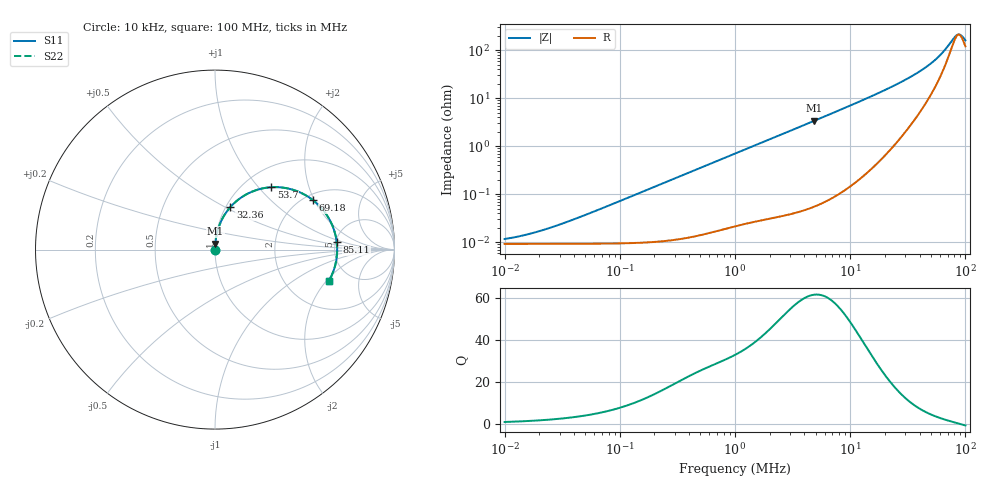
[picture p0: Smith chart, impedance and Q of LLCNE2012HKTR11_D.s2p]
! LLCNE2012HKTR11_D  S-PARAMETER MODEL  ( Standard Model )
! Model Generated by TAIYO YUDEN Corporation (http://www.ty-top.com)
! Version 1.0
! TAIYO YUDEN Control No. 210402
! Copyright(c) 2021 TAIYO YUDEN CO.,LTD. All Rights Reserved.
! Product Description (link to TY-COMPAS)
! https://ds.yuden.co.jp/TYCOMPAS/or/detail?pn=LLCNE2012HKTR11MD&u=M
! Products Name : Inductors
! Characteristics :
!  Inductance : 0.11 [uH] , SRF(min) : - [Hz] , DC Resistance(max) : 12 [mOhm]
!  Rated Current : Saturation  6.9 [A] (dL = 30 [%]), Temp Rise  5.8 [A] (dT = 40 [degC])
!  Case Size : 2.0 x 1.25 / 0.079 x 0.049 [mm/inch] , Thickness : 0.8 / 0.031 [mm/inch]
!  (Conditions: Temperature = 25 [degC] , DC Bias Current = 0 [A])
! External Node Assignments :
!  1  o---GGG---o  2
! GND o---------o GND
! Frequency Range : 10kHz  -  100MHz  [ 402 STEP ]
# MHz S RI R 50
! Freq[MHz].  S11 Real  S11 Imag  S21 Real  S21 Imag  S12 Real  S12 Imag  S22 Real  S22 Imag
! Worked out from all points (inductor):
!   401 points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, 10 kHz to 100 MHz, reference 50 ohm
!   read as one part in series: L = 113 nH near 38.91 kHz
!   highest Q = 61.6 at 4.898 MHz (marker M1), where L = 111 nH
!   self-resonance near 87.6 MHz
!   S11 on the Smith chart (normalised r, x): 10 kHz: 1.00, +0.00; 32.36 MHz: 1.05, +0.53; 53.7 MHz: 1.32, +1.17; 69.18 MHz: 2.22, +1.95; 85.11 MHz: 5.12, +0.78; 100 MHz: 3.41, -2.13
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0.01  9.2e-05 7.13e-05  0.9999 -7.13e-05  0.9999 -7.13e-05  9.2e-05 7.13e-05
0.013804  9.2e-05 9.84e-05  0.9999 -9.84e-05  0.9999 -9.84e-05  9.2e-05 9.84e-05
0.019953  9.21e-05 0.000142  0.9999 -0.000142  0.9999 -0.000142  9.21e-05 0.000142
0.029512  9.22e-05 0.00021  0.9999 -0.00021  0.9999 -0.00021  9.22e-05 0.00021
0.046774  9.26e-05 0.000333  0.9999 -0.000333  0.9999 -0.000333  9.26e-05 0.000333
0.218776  0.000105 0.00156  0.9999 -0.00156  0.9999 -0.00156  0.000105 0.00156
1  0.000263 0.00701  0.9997 -0.00701  0.9997 -0.00701  0.000263 0.00701
4.677351  0.00158 0.0324  0.9984 -0.0324  0.9984 -0.0324  0.00158 0.0324
4.897788  0.00171 0.0339  0.9983 -0.0339  0.9983 -0.0339  0.00171 0.0339
11.48154  0.00837 0.0803  0.9916 -0.0803  0.9916 -0.0803  0.00837 0.0803
21.87762  0.0335 0.1571  0.9665 -0.1571  0.9665 -0.1571  0.0335 0.1571
32.35937  0.0855 0.2369  0.9145 -0.2369  0.9145 -0.2369  0.0855 0.2369
42.65795  0.1733 0.307  0.8267 -0.307  0.8267 -0.307  0.1733 0.307
47.86301  0.2335 0.3327  0.7665 -0.3327  0.7665 -0.3327  0.2335 0.3327
53.70318  0.3129 0.3475  0.6871 -0.3475  0.6871 -0.3475  0.3129 0.3475
61.6595  0.4339 0.3335  0.5661 -0.3335  0.5661 -0.3335  0.4339 0.3335
69.1831  0.5456 0.2759  0.4544 -0.2759  0.4544 -0.2759  0.5456 0.2759
77.62471  0.6402 0.1635  0.3598 -0.1635  0.3598 -0.1635  0.6402 0.1635
85.1138  0.6785 0.041  0.3215 -0.041  0.3215 -0.041  0.6785 0.041
91.20108  0.6762 -0.0575  0.3238 0.0575  0.3238 0.0575  0.6762 -0.0575
95.49926  0.6597 -0.1203  0.3403 0.1203  0.3403 0.1203  0.6597 -0.1203
100  0.6327 -0.1775  0.3673 0.1775  0.3673 0.1775  0.6327 -0.1775
